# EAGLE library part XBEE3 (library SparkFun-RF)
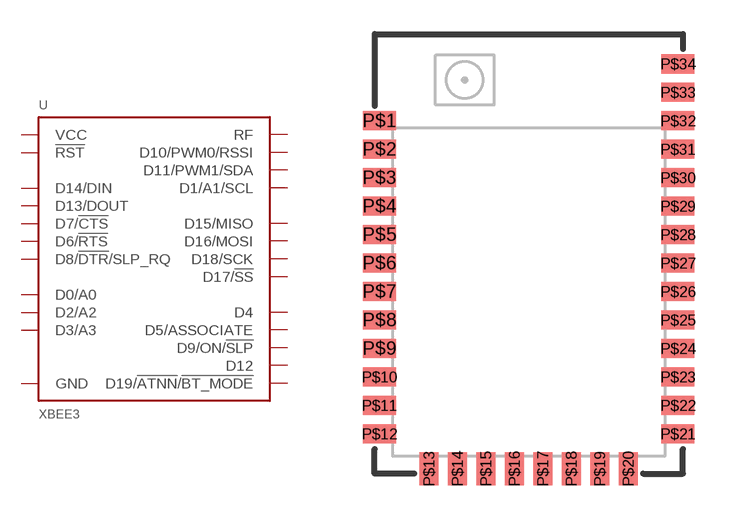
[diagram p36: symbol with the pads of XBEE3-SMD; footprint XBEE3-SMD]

Designator prefix U

## XBEE3 (PROD_ID: WRL-14444/ WRL-14467; VALUE: XBEE3_Micro)  [XBEE3-SMD]
P$1  GND
P$2  VCC
P$3  D13/DOUT
P$4  D14/DIN
P$5  D12
P$6  !RST  in
P$7  D10/PWM0/RSSI
P$8  D11/PWM1/SDA
P$9  D8/!DTR!/SLP_RQ
P$10  GND
P$11  D19/!ATNN!/!BT_MODE
P$12  GND
P$13  D18/SCK
P$14  D17/!SS
P$15  D16/MOSI
P$16  D15/MISO
P$21  GND
P$23  D4
P$24  D7/!CTS
P$25  D9/ON/!SLP
P$26  D5/ASSOCIATE
P$27  D6/!RTS
P$28  D3/A3
P$29  D2/A2
P$30  D1/A1/SCL
P$31  D0/A0
P$32  GND
P$33  RF
P$34  GND

## Footprint XBEE3-SMD (pad centres in mm)
smd 1.448 x 0.838: P$1 -6.553,5.847; P$2 -6.553,4.597; P$3 -6.553,3.348; P$4 -6.553,2.098; P$5 -6.553,0.848; P$6 -6.553,-0.401; P$7 -6.553,-1.651; P$8 -6.553,-2.901; P$9 -6.553,-4.15; P$10 -6.553,-5.4; P$11 -6.553,-6.65; P$12 -6.553,-7.899; P$21 6.553,-7.899; P$22 6.553,-6.65; P$23 6.553,-5.4; P$24 6.553,-4.15; P$25 6.553,-2.901; P$26 6.553,-1.651; P$27 6.553,-0.401; P$28 6.553,0.848; P$29 6.553,2.098; P$30 6.553,3.348; P$31 6.553,4.597; P$32 6.553,5.847; P$33 6.553,7.097; P$34 6.553,8.346
smd 0.838 x 1.448: P$13 -4.381,-9.436; P$14 -3.132,-9.436; P$15 -1.882,-9.436; P$16 -0.632,-9.436; P$17 0.617,-9.436; P$18 1.867,-9.436; P$19 3.117,-9.436; P$20 4.366,-9.436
